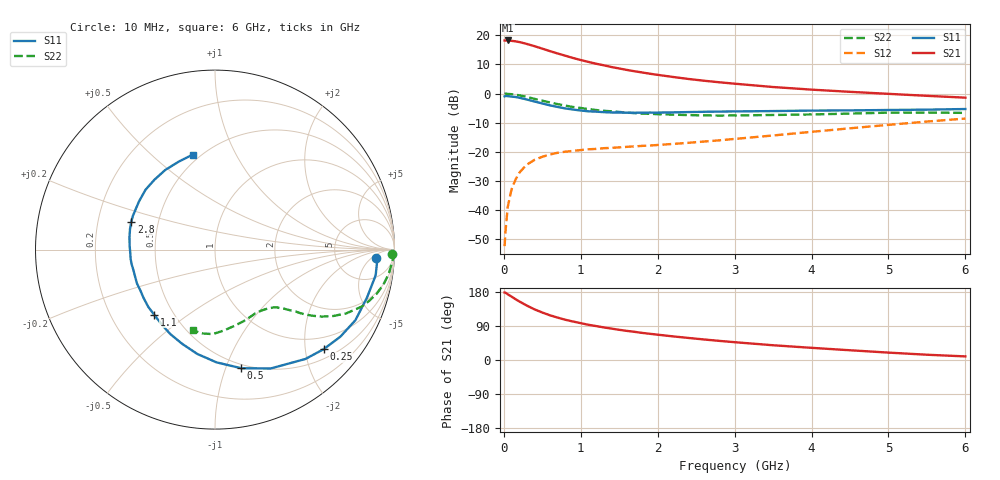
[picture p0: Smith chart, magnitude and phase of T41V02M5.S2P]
! Infineon Technologies  Discrete & RF Semiconductors
! BFR182T
! Si NPN RF Bipolar Junction Transistor in SC75
! VCE = 1 V  IC = 2.5 mA
! Common Emitter S-Parameters:  October  1999
# GHz  S  MA  R  50
!  f  S11  S21  S12  S22
! GHz  MAG  ANG  MAG  ANG  MAG  ANG  MAG  ANG
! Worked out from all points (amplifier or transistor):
!   36 points, 10 MHz to 6 GHz, reference 50 ohm
!   highest |S21| = 18.3 dB at 50 MHz (marker M1)
!   |S21| within 3 dB of that: start of sweep to 521.4 MHz
!   unconditionally stable (mu >= 1): 1.73 GHz to 4.578 GHz
!   at 250 MHz: K = 0.18, MSG = 21.6 dB, |S12| = -25.7 dB
!   at 1.4 GHz: K = 0.87, MSG = 13.9 dB, |S12| = -18.6 dB
!   at 6 GHz: K = 0.90, MSG = 3.6 dB, |S12| = -8.6 dB
!   S11 on the Smith chart (normalised r, x): 10 MHz: 15, -7; 250 MHz: 0.70, -2.39; 500 MHz: 0.46, -1.13; 1.1 GHz: 0.39, -0.38; 2.8 GHz: 0.35, +0.14; 6 GHz: 0.46, +0.69
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0.01  0.8958 -2.9  8.149 178.1  0.0024 87.2  0.9875 -1.5
0.02  0.9073 -2.3  8.165 177.8  0.0041 91.8  1 -1.7
0.05  0.9065 -9.1  8.181 173.5  0.0112 88.6  0.9896 -4.0
0.1  0.8881 -17.5  8.058 167.3  0.0227 81.4  0.9776 -7.9
0.15  0.8756 -26.7  7.909 160.7  0.033 75.2  0.9584 -11.7
0.2  0.8504 -34.8  7.688 154.7  0.0435 71.7  0.9349 -15.1
0.25  0.8212 -42.5  7.405 149.0  0.0517 67.0  0.9061 -18.3
0.3  0.7908 -50.4  7.118 143.5  0.0604 64.0  0.8773 -21.2
0.4  0.7314 -64.9  6.519 133.5  0.073 57.5  0.8133 -25.9
0.5  0.677 -77.5  5.915 125.3  0.0822 52.7  0.756 -29.3
0.6  0.6284 -89.2  5.361 117.9  0.0902 48.7  0.7041 -32.0
0.8  0.5563 -109.1  4.47 106.2  0.1006 44.0  0.6223 -35.6
0.9  0.5324 -117.9  4.089 101.5  0.1039 42.6  0.5897 -36.8
1.1  0.4966 -133.1  3.505 92.9  0.1107 41.0  0.5431 -38.7
1.3  0.4803 -146.1  3.061 86.0  0.1156 40.6  0.507 -40.5
1.6  0.4697 -161.8  2.55 76.8  0.1218 41.3  0.472 -43.0
2.2  0.4766 176.9  1.93 62.3  0.1368 45.4  0.4353 -49.7
2.8  0.4913 161.8  1.566 50.5  0.1576 49.7  0.4201 -57.9
3.5  0.5013 147.7  1.298 38.9  0.191 53.4  0.4295 -68.2
4.5  0.5152 130.9  1.073 25.7  0.2537 54.1  0.4537 -83.9
5.5  0.5303 112.3  0.916 13.9  0.3313 50.9  0.4722 -98.5
6  0.5437 103.2  0.852 9.5  0.373 47.6  0.4669 -105.2
